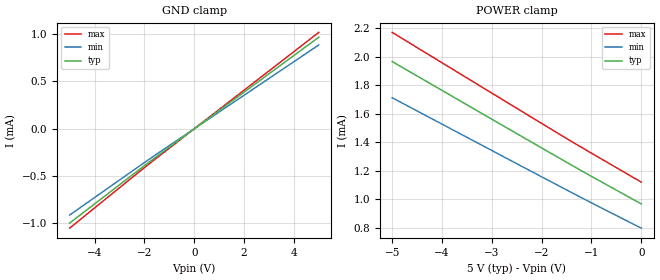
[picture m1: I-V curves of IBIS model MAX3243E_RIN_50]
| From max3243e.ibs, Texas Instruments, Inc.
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[Model]   MAX3243E_RIN_50
Model_type  Input
Vinl=0.8
Vinh=2.4
| variable   typ   min   max
C_comp   1.00pF   1.00pF   1.00pF
[Temperature Range]   40   100   -40
| Ambient temperature   25   85   -40
[Voltage range]   5   4.5   5.5
[GND Clamp]
| MAX3243E_RIN_50
|   Voltage   I(typ)   I(min)   I(max)
-5V       -995.8uA   -911.1uA   -1.049mA
-1.745V   -338.9uA   -310.3uA   -356.9uA
-435mV    -84.15uA   -77.05uA   -88.58uA
5V        967.2uA    885.6uA    1.018mA
[POWER Clamp]
| MAX3243E_RIN_50
|   Voltage   I(typ)   I(min)   I(max)
-5V       1.967mA    1.713mA    2.172mA
-1.515V   1.263mA    1.068mA    1.43mA
-915mV    1.144mA    959.2uA    1.306mA
-84.45fV  967.2uA    797uA      1.12mA
